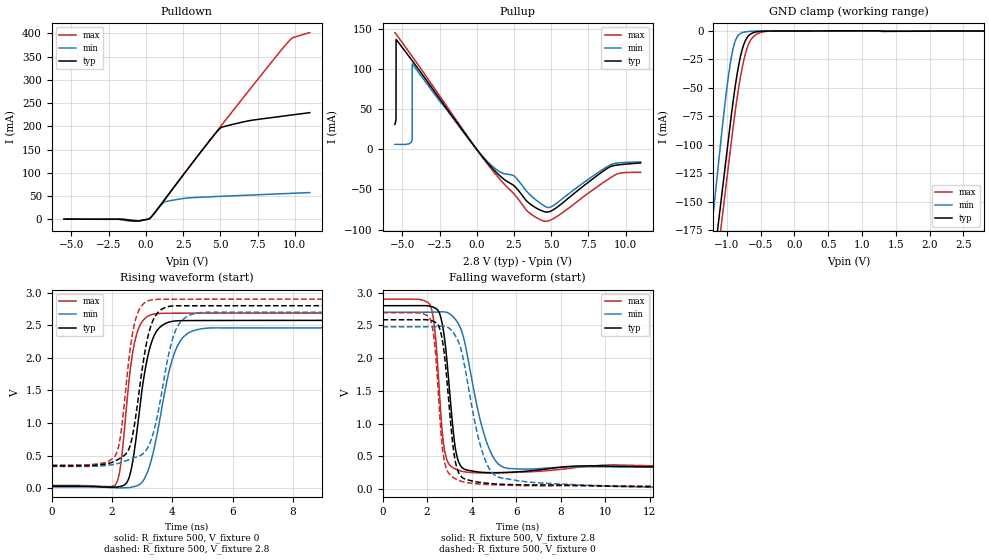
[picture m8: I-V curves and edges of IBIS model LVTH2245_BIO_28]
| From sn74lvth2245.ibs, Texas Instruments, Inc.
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[Model]   LVTH2245_BIO_28
Model_type  I/O
Vinl = 0.8
Vinh = 2.0
Enable   Active-Low
Vref =   0
Rref =   500
Cref =   50p
Vmeas =   1.5
| variable   typ   min   max
C_comp   6.56pF   5.40pF   8.58pF
| C_pullup   5.19pF   3.91pF   6.39pF
| C_pulldown   4.89pF   0.64pF   8.14pF
| C_tri-state   6.56pF   5.40pF   8.58pF
[Temperature Range]   40   -40   100
| Ambient temperature   25   -40   85
[Voltage range]   2.8   2.7   2.9
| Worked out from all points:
|   slope of the pulldown table from 0 to 0.42 V, typ, clamps not added: 52.5 ohm
|   slope of the pullup table from 0 to 0.42 V, typ, clamps not added: 42.2 ohm
|   GND clamp passes 1 mA (typ) near -0.58 V on its own axis
|   rising waveform, R_fixture 500, V_fixture 0: 20-80 % time 477ps typ, 654ps min, 373ps max; typ from 0.03 V to 2.58 V
|   falling waveform, R_fixture 500, V_fixture 2.8: 20-80 % time 411ps typ, 890ps min, 328ps max; typ from 2.8 V to 0.342 V
|   rising waveform, R_fixture 500, V_fixture 2.8: 20-80 % time 491ps typ, 627ps min, 388ps max; typ from 0.343 V to 2.8 V
|   falling waveform, R_fixture 500, V_fixture 0: 20-80 % time 441ps typ, 915ps min, 354ps max; typ from 2.58 V to 0.03 V
[GND Clamp]
| LVTH2245_BIO_28
|   Voltage   I(typ)   I(min)   I(max)
-5.5V     -2.567A    -2.796A    -2.573A
-1.235V   -223mA     -179.3mA   -245.7mA
-1.205V   -208.1mA   -162.2mA   -230.8mA
-1.15V    -180.8mA   -130.9mA   -203.6mA
-1.075V   -143.6mA   -88.6mA    -166.6mA
-975mV    -93.99mA   -38.62mA   -117.3mA
-900mV    -58.39mA   -13.38mA   -81.04mA
-825mV    -29.84mA   -3.359mA   -49.46mA
-775mV    -16.63mA   -1.489mA   -32.68mA
-650mV    -2.72mA    -290.9uA   -8.186mA
-375mV    -80.15uA   -70.16uA   -165.1uA
2.8V      31pA       23.95pA    -467.9pA
[Pulldown]
| LVTH2245_BIO_28
|   Voltage   I(typ)   I(min)   I(max)
-5.5V     844uA      863uA      652uA
-1.995V   608.7uA    951.5uA    511.8uA
-700mV    -3.18mA    -3.914mA   -2.193mA
260mV     2.161mA    2.307mA    2.135mA
1.28V     43.76mA    38.22mA    43.47mA
2.86V     110.8mA    46.42mA    111mA
4.465V    177mA      48.93mA    177.5mA
5.04V     197.5mA    49.75mA    201.1mA
6.985V    212.7mA    52.46mA    280.2mA
9.62V     224mA      56.02mA    384.2mA
9.9V      225.2mA    56.4mA     391.2mA
11V       229.7mA    57.86mA    401.9mA
[Pullup]
| LVTH2245_BIO_28
|   Voltage   I(typ)   I(min)   I(max)
-5.5V     31.12mA    6.38mA     145.9mA
-5.42V    38.45mA    6.361mA    143.9mA
-5.415V   137.3mA    6.36mA     143.8mA
-4.345V   111.1mA    11.68mA    116.4mA
-4.335V   110.9mA    13.39mA    116.1mA
-4.33V    110.7mA    106.8mA    116mA
495mV     -11.68mA   -10.71mA   -12.71mA
2.53V     -45.81mA   -33.56mA   -56.14mA
4.08V     -74.07mA   -64.61mA   -85.96mA
4.935V    -77.3mA    -72.14mA   -88.32mA
8.915V    -21.89mA   -19.8mA    -36.12mA
11V       -16.9mA    -15.57mA   -28.53mA
[Ramp]
| LVTH2245_BIO_28
| variable   typ   min   max
dV/dt_r   1.54/4.92E-10   1.47/6.61E-10   1.60/3.79E-10
dV/dt_f   1.53/4.33E-10   1.44/9.20E-10   1.59/3.53E-10
R_load = 500
[Rising Waveform]
| LVTH2245_BIO_28
R_fixture =   500
C_fixture =   0
L_fixture =   0
V_fixture =   0
V_fixture_min = 0
V_fixture_max = 0
|   Time   V(typ)   V(min)   V(max)
0s        30.33mV    18.78mV    42.49mV
2.105ns   16.21mV    5.695mV    46.89mV
2.285ns   27.77mV    4.553mV    348.4mV
2.5ns     92.51mV    6.886mV    1.344V
2.855ns   973.3mV    42.61mV    2.416V
3.155ns   1.951V     220.8mV    2.628V
3.475ns   2.404V     777.9mV    2.677V
4.15ns    2.567V     2.16V      2.684V
5.155ns   2.572V     2.455V     2.685V
50ns      2.575V     2.461V     2.687V
[Falling Waveform]
| LVTH2245_BIO_28
R_fixture =   500
C_fixture =   0
L_fixture =   0
V_fixture =   2.8
V_fixture_min = 2.7
V_fixture_max = 2.9
|   Time   V(typ)   V(min)   V(max)
0s        2.8V       2.7V       2.9V
2.125ns   2.793V     2.701V     2.816V
2.33ns    2.769V     2.702V     2.478V
2.525ns   2.708V     2.704V     1.635V
2.87ns    2.037V     2.699V     467.9mV
3.28ns    604.8mV    2.588V     305.7mV
3.725ns   297.1mV    2.186V     261.1mV
4.67ns    252.4mV    722.2mV    247mV
5.64ns    255.5mV    315.3mV    251.5mV
50ns      342.4mV    332.8mV    352mV
[Rising Waveform]
| LVTH2245_BIO_28
R_fixture =   500
C_fixture =   0
L_fixture =   0
V_fixture =   2.8
V_fixture_min = 2.7
V_fixture_max = 2.9
|   Time   V(typ)   V(min)   V(max)
0s        343.2mV    333.4mV    352.8mV
2.105ns   416.8mV    368.8mV    491.4mV
2.285ns   464.4mV    390.4mV    810.9mV
2.5ns     547.5mV    426.5mV    1.72V
2.815ns   1.189V     478mV      2.638V
3.12ns    2.164V     573.3mV    2.855V
3.355ns   2.569V     822.1mV    2.892V
4.09ns    2.797V     2.397V     2.898V
4.945ns   2.798V     2.693V     2.899V
50ns      2.8V       2.7V       2.9V
[Falling Waveform]
| LVTH2245_BIO_28
R_fixture =   500
C_fixture =   0
L_fixture =   0
V_fixture =   0
V_fixture_min = 0
V_fixture_max = 0
|   Time   V(typ)   V(min)   V(max)
0s        2.585V     2.478V     2.693V
2.105ns   2.58V      2.479V     2.615V
2.315ns   2.557V     2.479V     2.291V
2.505ns   2.499V     2.482V     1.47V
2.86ns    1.781V     2.479V     318.2mV
3.285ns   394.2mV    2.332V     154.1mV
3.875ns   136.2mV    1.516V     94.77mV
4.82ns    85.31mV    298.1mV    67.9mV
6.56ns    63.95mV    107.1mV    51.51mV
50ns      30.32mV    18.74mV    42.51mV
